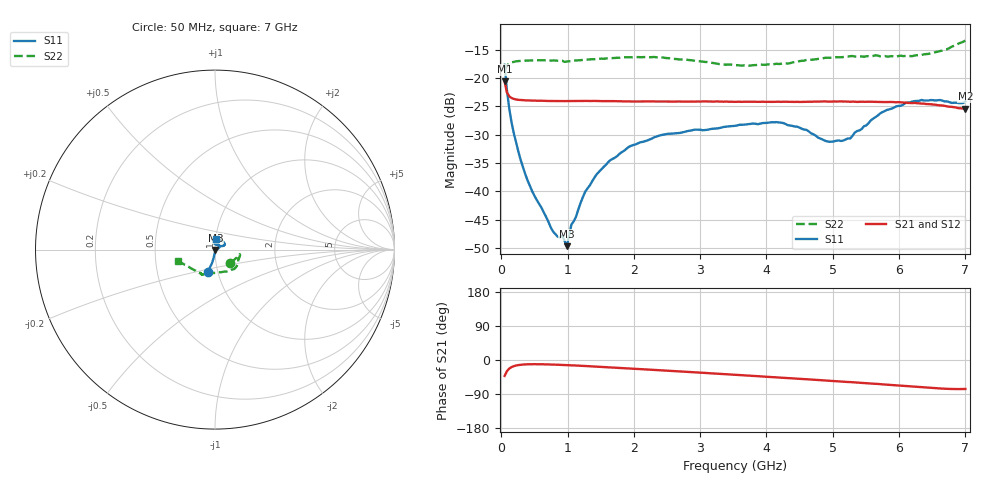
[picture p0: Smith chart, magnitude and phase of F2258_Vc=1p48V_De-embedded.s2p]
! Integrated Device Technology
! Corporate Headquarters
! 6024 Silver Creek Valley Road
! San Jose, CA 95138  USA
! Phone:  1-408-284-8200
! Toll Free:  1-800-223-1366
! Webpage:  http://www.idt.com/
! Timing and RF Division
! 515 Groton Road, Suite 102
! Westford, MA 01886-6024
! Device:  F2258
! Description: Voltage Variable RF Attenuator
! Frequency:  50.0 -  6000.00 MHz
! Package:  3x3 mm Thin QFN Plastic Package: 16 pin
! Ports:  2 RF, 2 DC
!  Pin  1  = NC
!  Pin  2  = NC
!  Pin  3  = RF2  = Port 2
!  Pin  4  = GND
!  Pin  5  = Vdd
!  Pin  6  = NC
!  Pin  7  = VCTRL
!  Pin  8  = NC
!  Pin  9  = GND
!  Pin 10  = RF1  = Port 1
!  Pin 11  = NC
!  Pin 12  = NC
!  Pin 13  = NC
!  Pin 14  = NC
!  Pin 15  = NC
!  Pin 16  = NC
! Vcntrl:  1.480 Volts
! Vdd:  +3.300 Volts
! Current:  1.165 mA
! Data:  The device was measured on a the F2258 evaluation board which has
!  individual transmission lines to the RF pins.  Data was collected
!  using a calibrated network analyzer.  The evaluation board was
!  de-embedded using a TRL calibration technique.
!  The reference plane is the edge of the package pin.
! Misc:  SN 10
!  Action Tracker AT0285
! Date Measured:  2014-12-10
! Date:  2016-01-13  MJV
! Note:
!  Integrated Device Technology supplies this data as a sample of measured
!  data at the package pin for this product.  Your particular data for this
!  product may vary.
!  Data was taken at 25 degrees C.
!  Integrated Device Technology reserves the right to change this data at anytime.
!Freq_(GHz)  S11M_(dB)  S11P_(deg)  S21M_(dB)  S21P_(deg)  S12M_(dB)  S12P_(deg)  S22M_(dB)  S22P_(deg)
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# GHz S dB R 50
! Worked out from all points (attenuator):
!   201 points, 50 MHz to 7 GHz, reference 50 ohm
!   highest |S21| = -20.63 dB at 50 MHz (marker M1); lowest = -25.4 dB at 7 GHz (marker M2)
!   lowest |S11| = -49.7 dB at 988.2 MHz (marker M3), VSWR 1.01, Z = 50.2 - j0.219 ohm
!   |S11| at or under -10 dB: start of sweep to end of sweep
!   |S22| runs from -18.9 to -13.4 dB; largest |S21 - S12| = 0.00072
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0.05  -17.68 -107.8  -20.63 -42.0  -20.62 -42.0  -18.85 -41.2
0.08475  -22.16 -102.6  -22.57 -29.5  -22.57 -29.5  -17.86 -21.0
0.15425  -27.83 -99.1  -23.54 -18.7  -23.54 -18.7  -17.26 -12.8
0.2585  -33.03 -95.8  -23.86 -13.4  -23.87 -13.4  -17.03 -10.5
0.36275  -37.00 -92.2  -23.96 -11.6  -23.96 -11.6  -16.96 -11.0
0.77975  -47.07 -48.3  -24.07 -12.1  -24.08 -12.1  -16.92 -17.4
0.91875  -47.77 -6.5  -24.08 -13.0  -24.08 -13.0  -16.97 -20.5
0.98825  -49.66 -41.4  -24.08 -13.5  -24.09 -13.5  -17.12 -21.5
1.05775  -45.83 -15.0  -24.07 -14.0  -24.10 -14.0  -17.02 -22.6
1.2315  -40.99 5.5  -24.07 -15.5  -24.08 -15.5  -16.83 -25.8
1.44  -36.97 11.0  -24.07 -17.6  -24.09 -17.6  -16.69 -29.5
1.6485  -34.47 16.1  -24.10 -19.7  -24.10 -19.6  -16.52 -33.1
1.9265  -32.14 25.0  -24.15 -22.4  -24.14 -22.4  -16.38 -37.7
2.37825  -30.19 36.6  -24.16 -26.9  -24.18 -26.9  -16.37 -45.5
3.525  -28.45 86.2  -24.22 -39.0  -24.18 -39.0  -17.75 -77.2
4.1505  -27.80 103.0  -24.22 -45.8  -24.18 -45.9  -17.51 -99.4
4.7065  -29.94 93.0  -24.19 -52.0  -24.21 -51.9  -16.77 -110.6
4.94975  -31.27 75.0  -24.19 -54.7  -24.24 -54.6  -16.45 -113.1
5.2625  -30.69 45.9  -24.20 -58.3  -24.26 -58.2  -16.17 -115.6
5.85325  -25.54 24.4  -24.25 -65.6  -24.32 -65.5  -16.22 -120.6
6.33975  -23.89 31.1  -24.53 -72.0  -24.59 -72.0  -15.96 -132.7
7  -24.15 83.5  -25.43 -76.4  -25.50 -76.4  -13.40 -163.3
